(* Logix 5000 AddOnInstructionDefinition export B256_SUB; software revision 30.00 *)

ADD_ON_INSTRUCTION B256_ADD   (* revision 1.0 20170916, vendor Kenneth A. Fischer *)
// c3=c1+c2 with no reduction
// Revision note:
// Rev1.0: 20170916 - Initial Release
VAR_IN_OUT
   Inp_C1 : DINT[22]; {required}
   Inp_C2 : DINT[22]; {required}
   Out_C3 : DINT[22]; {required}
END_VAR
VAR
   i : INT;
END_VAR

ROUTINE Logic   (* ladder *)
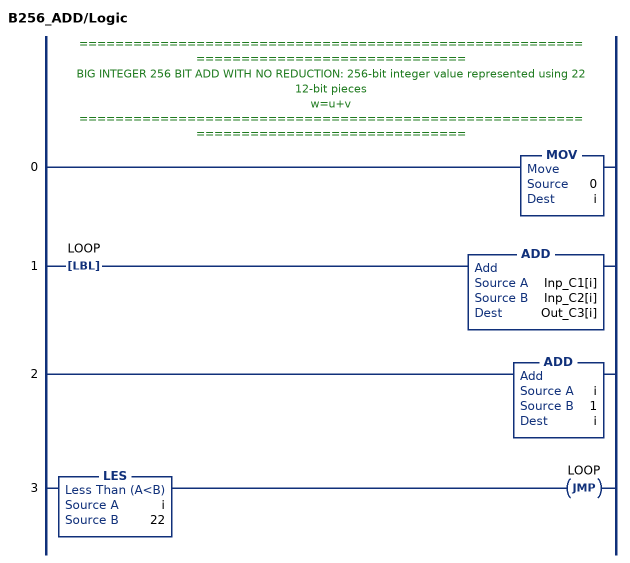
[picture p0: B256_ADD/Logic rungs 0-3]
   // ======================================================================================
   // BIG INTEGER 256 BIT ADD WITH NO REDUCTION: 256-bit integer value represented using 22 12-bit pieces
   // w=u+v
   // ======================================================================================
   0: MOV(0,i);
   1: LBL(LOOP)ADD(Inp_C1[i],Inp_C2[i],Out_C3[i]);
   2: ADD(i,1,i);
   3: LES(i,22)JMP(LOOP);
END_ROUTINE
END_ADD_ON_INSTRUCTION

ADD_ON_INSTRUCTION D_SHR   (* revision 1.0, vendor Ken Fischer, NSWCPD, C512 *)
// DINT bit shift right of the 32-bit argument Inp_A by Inp_B bits with paddding by zeros on the right
// Revision note:
// Rev1.0: TBD - Initial Release
VAR_IN_OUT
   Inp_A : DINT; {required}   // 64-bit Integer to be right circular rotated
END_VAR
VAR_INPUT
   Inp_B : INT; {required}   // Number of bits to shift
END_VAR
VAR_IN_OUT
   Out : DINT; {required}   // Result
END_VAR
VAR
   BSR_Cntrl : CONTROL := (LEN := 32);
   ONS : BOOL;
   Source_Bit : BOOL;
   Wrk_InpA : DINT[2];
END_VAR

ROUTINE Logic   (* ladder *)
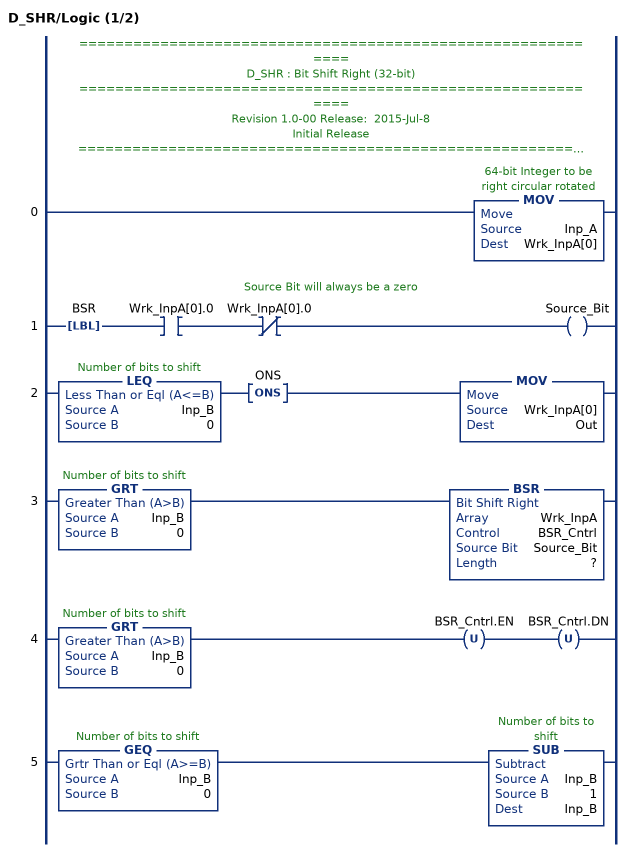
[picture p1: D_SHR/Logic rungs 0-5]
   // ============================================================
   // D_SHR : Bit Shift Right (32-bit)
   // ============================================================
   // Revision 1.0-00 Release:  2015-Jul-8
   // Initial Release
   // ============================================================
   // Performs a right bit shift of the 32-bit argument Inp_A by the
   // number of bits defined in the 16-bit argument Inp_B, with padding by zeros.
   0: MOV(Inp_A,Wrk_InpA[0]);
   // Source Bit will always be a zero
   1: LBL(BSR)XIC(Wrk_InpA[0].0)XIO(Wrk_InpA[0].0)OTE(Source_Bit);
   2: LEQ(Inp_B,0)ONS(ONS)MOV(Wrk_InpA[0],Out);
   3: GRT(Inp_B,0)BSR(Wrk_InpA,BSR_Cntrl,Source_Bit,?);
   4: GRT(Inp_B,0)OTU(BSR_Cntrl.EN)OTU(BSR_Cntrl.DN);
   5: GEQ(Inp_B,0)SUB(Inp_B,1,Inp_B);
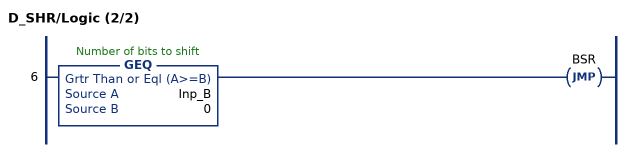
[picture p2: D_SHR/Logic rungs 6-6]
   6: GEQ(Inp_B,0)JMP(BSR);
END_ROUTINE
END_ADD_ON_INSTRUCTION

ADD_ON_INSTRUCTION B256_NRED   (* revision 1.0 20170916, vendor Kenneth A. Fischer *)
// Reduce 256-bit integer stored in 22 pieces by propagating carries
// Revision note:
// Rev1.0: 20170916 - Initial Release
VAR_IN_OUT
   Inp_C : DINT[22]; {required}
END_VAR
VAR
   D_SHR : D_SHR;
   temp : DINT;
   i : INT;
END_VAR

ROUTINE Logic   (* ladder *)
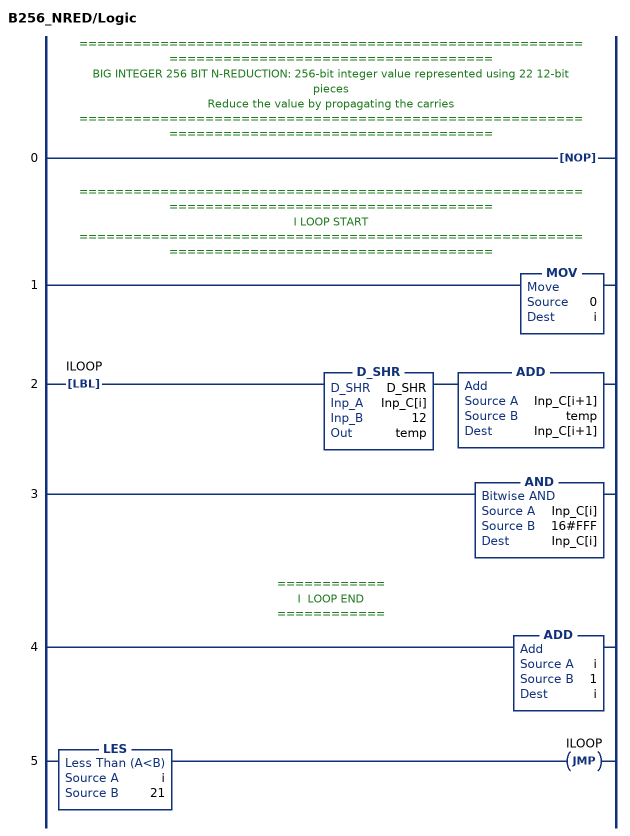
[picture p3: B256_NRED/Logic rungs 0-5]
   // ============================================================================================
   // BIG INTEGER 256 BIT N-REDUCTION: 256-bit integer value represented using 22 12-bit pieces
   // Reduce the value by propagating the carries
   // ============================================================================================
   0: NOP();
   // ============================================================================================
   // I LOOP START
   // ============================================================================================
   1: MOV(0,i);
   2: LBL(ILOOP)D_SHR(D_SHR,Inp_C[i],12,temp)ADD(Inp_C[i+1],temp,Inp_C[i+1]);
   3: AND(Inp_C[i],16#FFF,Inp_C[i]);
   // ============
   // I  LOOP END
   // ============
   4: ADD(i,1,i);
   5: LES(i,21)JMP(ILOOP);
END_ROUTINE
END_ADD_ON_INSTRUCTION

ADD_ON_INSTRUCTION B256_SUB   (* revision 1.0 20170916, vendor Kenneth A. Fischer *)
// c3=c1-c2 with reduction
// Revision note:
// Rev1.0: 20170916 - Initial Release
VAR_IN_OUT
   Inp_C1 : DINT[22]; {required}
   Inp_C2 : DINT[22]; {required}
   Out_C3 : DINT[22]; {required}
END_VAR
VAR
   B256_ADD : B256_ADD;
   B256_NRED : B256_NRED;
   temp : DINT;
   i : INT;
END_VAR

ROUTINE Logic   (* ladder *)
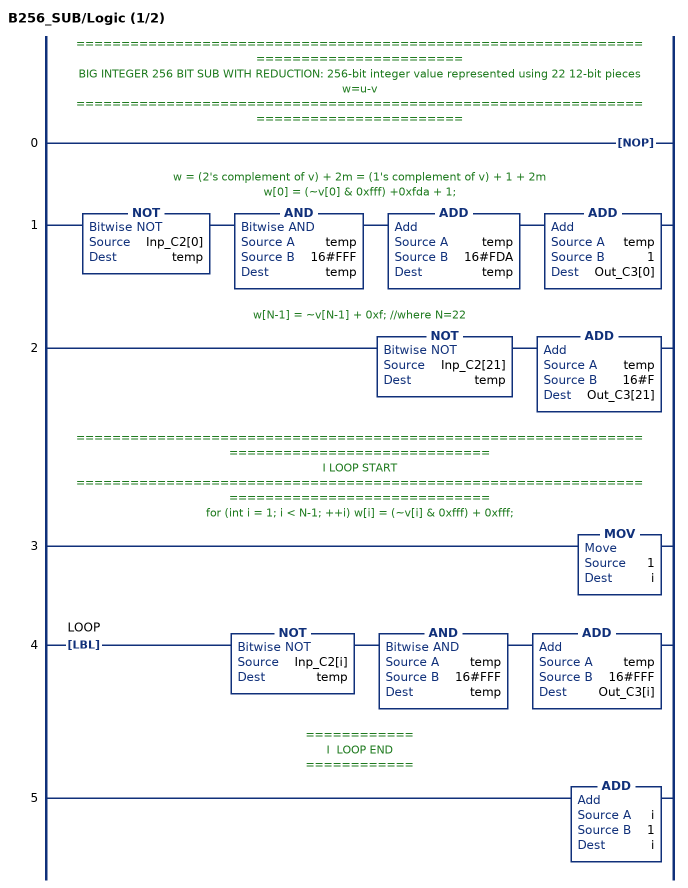
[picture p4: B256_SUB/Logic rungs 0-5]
   // ======================================================================================
   // BIG INTEGER 256 BIT SUB WITH REDUCTION: 256-bit integer value represented using 22 12-bit pieces
   //  w=u-v
   // ======================================================================================
   0: NOP();
   // w = (2's complement of v) + 2m = (1's complement of v) + 1 + 2m
   // w[0] = (~v[0] & 0xfff) +0xfda + 1;
   1: NOT(Inp_C2[0],temp)AND(temp,16#FFF,temp)ADD(temp,16#FDA,temp)ADD(temp,1,Out_C3[0]);
   // w[N-1] = ~v[N-1] + 0xf; //where N=22
   2: NOT(Inp_C2[21],temp)ADD(temp,16#F,Out_C3[21]);
   // ============================================================================================
   // I LOOP START
   // ============================================================================================
   // for (int i = 1; i < N-1; ++i) w[i] = (~v[i] & 0xfff) + 0xfff;
   3: MOV(1,i);
   4: LBL(LOOP)NOT(Inp_C2[i],temp)AND(temp,16#FFF,temp)ADD(temp,16#FFF,Out_C3[i]);
   // ============
   // I  LOOP END
   // ============
   5: ADD(i,1,i);
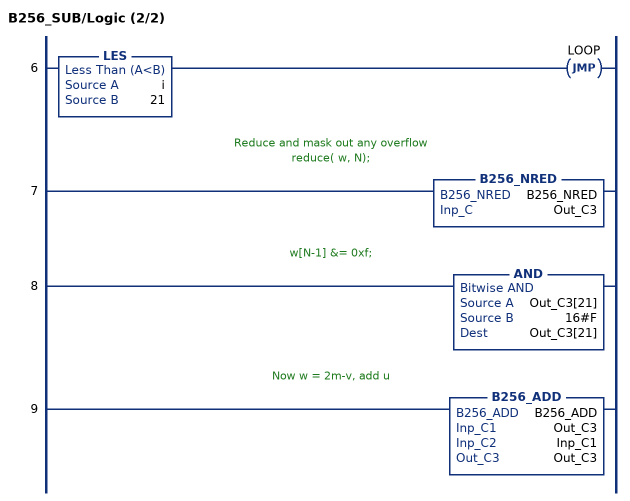
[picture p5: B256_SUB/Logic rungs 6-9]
   6: LES(i,21)JMP(LOOP);
   // Reduce and mask out any overflow
   // reduce( w, N);
   7: B256_NRED(B256_NRED,Out_C3);
   // w[N-1] &= 0xf;
   8: AND(Out_C3[21],16#F,Out_C3[21]);
   // Now w = 2m-v, add u
   9: B256_ADD(B256_ADD,Out_C3,Inp_C1,Out_C3);
END_ROUTINE
END_ADD_ON_INSTRUCTION
